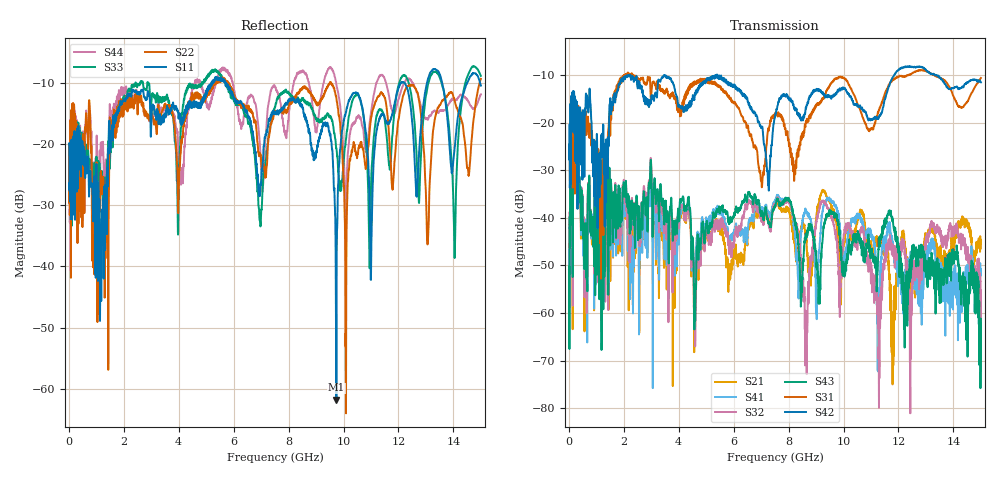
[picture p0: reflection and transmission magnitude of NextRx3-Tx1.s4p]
! FILE: N:\QM 2007\Prüfprotokolle\Highspeed\Konfektionierte Ltg\L45593-D106\D30\8216\0002\Next  Platine 2\NextRx3-Tx1.s4p
# MHz S DB R 50.00
! FREQ  S11  S12  S13  S14
!  S21  S22  S23  S24
!  S31  S32  S33  S34
!  S41  S42  S43  S44
!  DB  ANG  DB  ANG  DB  ANG  DB  ANG
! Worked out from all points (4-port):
!   2999 points, 10 MHz to 15 GHz, reference 50 ohm
!   strongest paths, dB at 10 MHz, 3.755 GHz, 7.505 GHz, 11.26 GHz, 15 GHz:
!     S42: -24.9, -11.4, -18.8, -19.2, -11.6
!     S31: -25.0, -14.5, -18.2, -17.9, -10.6
!     S43: -51.8, -39.9, -37.6, -49.0, -61.2
!     S32: -50.8, -48.7, -37.3, -59.7, -55.5
!     S41: -46.7, -42.6, -36.5, -72.2, -50.8
!     S21: -45.4, -48.7, -37.4, -45.8, -45.3
!   lowest |S11| = -61.7 dB at 9.74 GHz (marker M1), VSWR 1.00, Z = 50.1 - j0.0522 ohm
!   |S11| at or under -10 dB: start of sweep to 5.21 GHz; 5.697 GHz to 12.11 GHz (6.413 GHz wide, 72 % of centre); 13.59 GHz to 14.5 GHz (918 MHz wide, 6.54 % of centre)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
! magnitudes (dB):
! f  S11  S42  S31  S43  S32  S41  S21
! 10 MHz  -19.9  -24.9  -25.0  -51.8  -50.8  -46.7  -45.4
! 8.14 GHz  -12.9  -15.5  -27.4  -38.0  -39.2  -39.2  -41.9
! 8.635 GHz  -15.7  -17.1  -19.8  -44.4  -59.7  -38.4  -44.6
! 9.74 GHz  -61.7  -14.0  -10.7  -39.3  -44.4  -37.8  -41.3
! 10.07 GHz  -15.0  -13.2  -10.9  -50.5  -42.5  -48.2  -43.0
! 14.04 GHz  -20.9  -12.7  -14.9  -48.3  -42.4  -51.1  -44.6
! 15 GHz  -10.5  -11.6  -10.6  -61.2  -55.5  -50.8  -45.3
